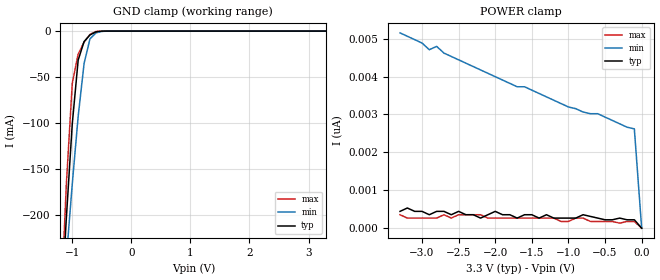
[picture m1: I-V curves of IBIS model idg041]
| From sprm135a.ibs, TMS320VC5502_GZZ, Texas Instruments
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[Model]   idg041
Model_type   Input
Polarity   Non-Inverting
| signals   A, Y
Vinl = 0.8V
Vinh = 2.0V
|   typ   min   max
C_comp   1.6514p   1.5581p   1.8632p
|   typ   min   max
[Temperature Range]   25   -40   125
|   typ   min   max
[Voltage Range]   3.30V   3.00V   3.60V
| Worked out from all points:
|   GND clamp passes 1 mA (typ) near -0.61 V on its own axis
[GND_clamp]
|   Voltage   I(typ)   I(min)   I(max)
-3.3V     -2.964A    -2.238A    -3.848A
-1.2V     -316.1mA   -330.3mA   -312mA
-1.1V     -202.7mA   -246.4mA   -166mA
-1V       -100.7mA   -165.9mA   -56.94mA
-900mV    -31.48mA   -92.52mA   -24.86mA
-800mV    -11.38mA   -35.13mA   -12.05mA
-700mV    -4.184mA   -8.441mA   -3.556mA
-600mV    -818.7uA   -2.03mA    -409.8uA
-500mV    -75.21uA   -364.5uA   -19.35uA
-400mV    -4.217uA   -44.76uA   -434.5nA
3.3V      222pA      2.753nA    133.2pA
[POWER_clamp]
|   Voltage   I(typ)   I(min)   I(max)
-3.3V     444.1pA    5.151nA    355.3pA
-3.2V     532.9pA    5.063nA    266.4pA
-2.9V     355.3pA    4.707nA    266.4pA
-2.8V     444.1pA    4.796nA    266.4pA
-2.6V     355.3pA    4.53nA     266.4pA
-2.5V     444.1pA    4.441nA    355.3pA
-2.2V     266.4pA    4.174nA    355.3pA
-2V       444.1pA    3.997nA    266.4pA
-1.7V     266.4pA    3.73nA     266.4pA
-800mV    355.3pA    3.064nA    266.4pA
-100mV    222pA      2.62nA     177.6pA
0V        1pA        1pA        1pA
